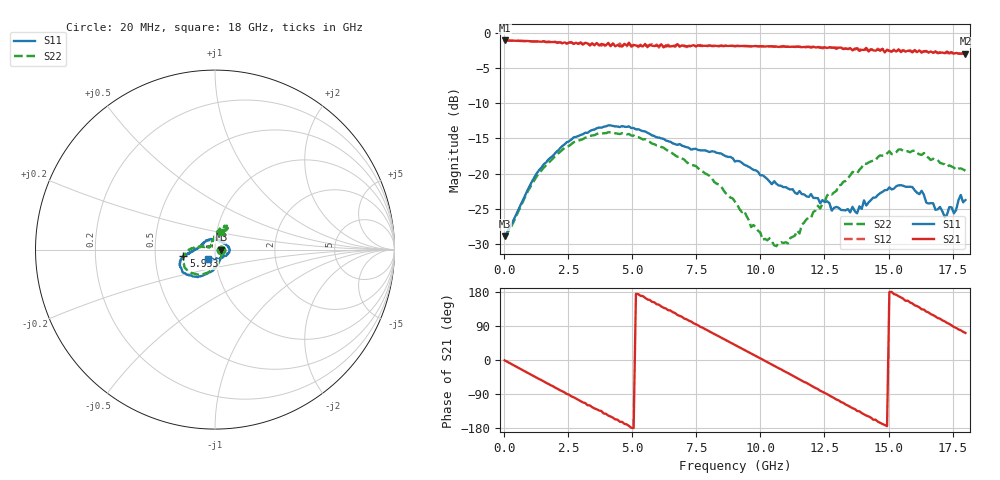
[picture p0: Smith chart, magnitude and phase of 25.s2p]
!Agilent Technologies,N5230A,US43500223,A.07.50.48
!Agilent N5230A: A.07.50.48
!Date: Sunday, January 17, 2016 15:24:19
!Correction: S11(Full 2 Port(1,2))
!S21(Full 2 Port(1,2))
!S12(Full 2 Port(1,2))
!S22(Full 2 Port(1,2))
!S2P File: Measurements: S11, S21, S12, S22:
# Hz S  RI  R 50
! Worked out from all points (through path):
!   201 points, 20 MHz to 18 GHz, reference 50 ohm
!   highest |S21| = -1.09 dB at 20 MHz (marker M1); lowest = -3.0 dB at 18 GHz (marker M2)
!   group delay of S21, straight-line fit = 99.6 ps
!   lowest |S11| = -29.0 dB at 20 MHz (marker M3), VSWR 1.07, Z = 53.7 - j0.123 ohm
!   |S11| at or under -10 dB: start of sweep to end of sweep
!   |S22| runs from -30.3 to -14.1 dB; largest |S21 - S12| = 0.042
!   S11 on the Smith chart (normalised r, x): 20 MHz: 1.07, -0.00; 5.953 GHz: 0.70, -0.05; 18 GHz: 0.92, -0.10
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2e7  0.0357 -0.00115  0.8817 -0.0132  0.882 -0.0128  0.0351 -0.00169
9.19e8  0.0197 -0.0738  0.7268 -0.4862  0.7245 -0.4873  0.0218 -0.0712
1.7281e9  -0.0224 -0.1237  0.3896 -0.7653  0.3901 -0.7749  -0.023 -0.1168
2.5372e9  -0.0814 -0.1485  -0.0223 -0.8533  -0.0167 -0.8497  -0.0766 -0.1371
3.0766e9  -0.1167 -0.15  -0.3086 -0.7635  -0.3128 -0.77  -0.1133 -0.1342
4.0655e9  -0.1788 -0.1275  -0.7101 -0.4639  -0.6907 -0.4759  -0.1673 -0.1031
4.8746e9  -0.1986 -0.0857  -0.8457 -0.0879  -0.8279 -0.0987  -0.1802 -0.0628
5.9534e9  -0.1768 -0.0373  -0.6806 0.4389  -0.6941 0.4466  -0.1578 -0.0137
6.0433e9  -0.1767 -0.035  -0.6661 0.451  -0.6396 0.4573  -0.1571 -0.0105
6.7625e9  -0.1578 -0.025  -0.4007 0.7255  -0.4056 0.7212  -0.1311 0.0082
7.6615e9  -0.1446 -0.0217  0.0359 0.8049  0.0468 0.8179  -0.1047 0.00991
9.01e9  -0.1214 -0.00887  0.6184 0.5146  0.6247 0.5051  -0.0613 0.0142
1.04484e10  -0.0829 0.0128  0.7838 -0.1685  0.7791 -0.1817  -0.0293 0.015
1.10777e10  -0.0736 0.0266  0.6554 -0.4511  0.652 -0.4603  -0.0203 0.0246
1.20666e10  -0.0435 0.051  0.2614 -0.7533  0.2533 -0.7488  -0.0112 0.0521
1.3505e10  0.0193 0.0494  -0.4329 -0.6472  -0.4258 -0.6367  0.0135 0.0961
1.41343e10  0.0484 0.0341  -0.6523 -0.4304  -0.6346 -0.4123  0.0249 0.1144
1.50333e10  0.0789 0.012  -0.7418 0.00669  -0.7468 0.0107  0.0541 0.1335
1.57525e10  0.0796 -0.012  -0.6833 0.2978  -0.6619 0.3258  0.0682 0.1267
1.66515e10  0.0483 -0.0382  -0.3794 0.6324  -0.3647 0.6362  0.0599 0.1093
1.71909e10  0.00685 -0.0488  -0.1494 0.7004  -0.1219 0.7091  0.0542 0.1029
1.8e10  -0.0382 -0.0523  0.2251 0.6738  0.2462 0.6605  0.0311 0.0999
